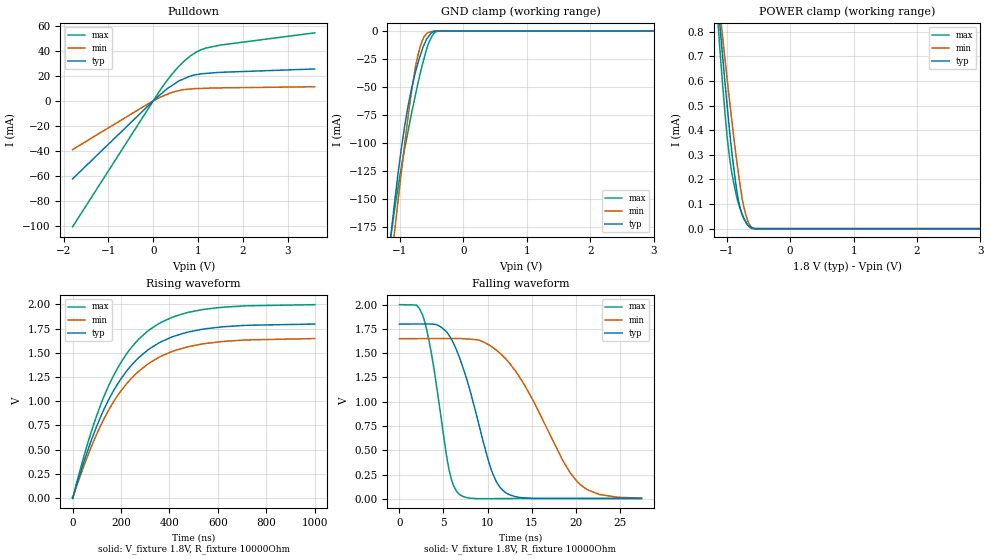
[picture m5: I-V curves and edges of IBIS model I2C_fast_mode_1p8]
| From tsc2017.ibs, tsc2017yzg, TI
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|   i2c_fast_mode_1p8 Model
[Model]   I2C_fast_mode_1p8
Model_type   I/O_open_drain
Polarity   Non-Inverting
Enable   Active-Low
Vinl = 0.54
Vinh = 1.26
Vmeas = 0.9
Vref = 1.8
Cref = 400pF
Rref = 10000
|   typ   min   max
|   (nom PVT)   (Fast PVT)   (slow PVT)
|Average
C_comp   1.636e-11   1.570e-11   1.694e-11
|ON state : BUFFER OUTPUT TURNED LOW
|C_comp   4.204e-11   3.525e-11   4.243e-11
|OFF state: BUFFER in HIGH IMPEDANCE
|C_comp   1.636e-11   1.570e-11   1.694e-11
|C_comp from frequency method(F=3.4MHz)
| Where nom  PVT is Nominal Process, 1.8V, 25C
|   Fast PVT is Strong Process,  2V, -40C
|   Slow PVT is Weak Process,   1.65V, 85C
[Model Spec]
Vinl   0.54   0.495   0.6
Vinh   1.26   1.155   1.4
[Voltage Range]   1.8   1.65   2
|Ambient Temperature   25   85   -40
|Junction Temperature
[Temperature Range]   25   85   -40
[Pullup Reference]   1.8   1.65   2
[Pulldown Reference]   0   0   0
[Power Clamp Reference]   1.8   1.65   2
[GND Clamp Reference]   0   0   0
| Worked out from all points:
|   slope of the pulldown table from 0 to 0.27 V, typ, clamps not added: 32 ohm
|   GND clamp passes 1 mA (typ) near -0.48 V on its own axis
|   POWER clamp passes 1 mA (typ) near -1.17 V on its own axis
|   falling waveform, V_fixture 1.8V, R_fixture 10000Ohm: 20-80 % time 3.32ns typ, 5.8ns min, 2ns max; typ from 1.8 V to 0.005 V
|   rising waveform, V_fixture 1.8V, R_fixture 10000Ohm: 20-80 % time 223ns typ, 231ns min, 214ns max; typ from 0.005 V to 1.8 V
[Pulldown]
|   Voltage   I(typ)   I(min)   I(max)
-1.8V     -62.32mA   -38.9mA    -100.6mA
-102.2mV  -3.57mA    -2.096mA   -5.745mA
142mV     4.543mA    2.624mA    7.89mA
428mV     12.49mA    6.872mA    21.76mA
577.8mV   15.99mA    8.178mA    27.78mA
828mV     19.82mA    9.449mA    35.86mA
1.064V    21.55mA    9.913mA    40.79mA
1.498V    22.77mA    10.34mA    44.52mA
3.6V      25.44mA    11.26mA    54.29mA
[GND Clamp]
|   Voltage   I(typ)   I(min)   I(max)
-1.8V     -554.1mA   -567.1mA   -560.8mA
-1.15V    -186.5mA   -213.7mA   -186.5mA
-1.085V   -153.9mA   -180mA     -160.5mA
-1.076V   -149.4mA   -175.2mA   -156.7mA
-925.2mV  -84.72mA   -101.1mA   -105.1mA
-856.2mV  -62.68mA   -69.86mA   -85.05mA
-757.2mV  -37.1mA    -32.55mA   -57.67mA
-656.5mV  -18.02mA   -9.927mA   -32.4mA
-570.7mV  -6.514mA   -1.785mA   -14.58mA
-468mV    -361.9uA   0A         -2.378mA
-388mV    0A         0A         0A
3.6V      0A         0A         0A
[POWER Clamp]
|   Voltage   I(typ)   I(min)   I(max)
-1.8V     2.967mA    2.622mA    3.431mA
-1.13V    891.2uA    937uA      808.9uA
-1.106V   819.6uA    877.5uA    720.8uA
-1.064V   696.2uA    775.3uA    582.1uA
-998mV    511.7uA    618uA      382.4uA
-926mV    325.3uA    452.4uA    236.2uA
-862.2mV  192uA      313.9uA    150.3uA
-806.4mV  103uA      206.5uA    94.43uA
-727.5mV  40.37uA    84.06uA    40.29uA
-638mV    9.164uA    15.43uA    4.889uA
-570.7mV  1.367uA    0A         0A
3.6V      0A         0A         0A
[Ramp]
R_load = 10000
|   typ   min   max
dV/dt_r   1.07565/2.23183e-07   0.983656/2.30409e-07   1.1969/2.14093e-07
dV/dt_f   1.0769/3.31864e-09   0.985092/5.77252e-09   1.19792/2.00039e-09
[Falling Waveform]
V_fixture = 1.8V
V_fixture_min = 1.65V
V_fixture_max = 2V
R_fixture = 10000Ohm
|   Time   V(typ)   V(min)   V(max)
0s        1.8V       1.65V      2V
1.925ns   1.801V     1.65V      1.996V
2.7ns     1.801V     1.65V      1.876V
3.725ns   1.799V     1.65V      1.448V
5.625ns   1.685V     1.651V     303mV
6.85ns    1.446V     1.651V     43.86mV
10.4ns    304.8mV    1.571V     1.68mV
12.08ns   62.28mV    1.44V      2.856mV
20.23ns   4.394mV    171mV      3.526mV
27.45ns   5.294mV    6.823mV    3.458mV
[Rising Waveform]
V_fixture = 1.8V
V_fixture_min = 1.65V
V_fixture_max = 2V
R_fixture = 10000Ohm
|   Time   V(typ)   V(min)   V(max)
0s        5.166mV    8.172mV    3.46mV
78.45ns   601.9mV    534.8mV    692.6mV
112ns     815.3mV    726.6mV    935.6mV
145.7ns   998.5mV    892.4mV    1.141V
222.8ns   1.31V      1.179V     1.488V
309ns     1.525V     1.38V      1.721V
407.2ns   1.661V     1.51V      1.863V
533.1ns   1.742V     1.59V      1.946V
705.6ns   1.783V     1.632V     1.985V
1us       1.798V     1.648V     1.998V
